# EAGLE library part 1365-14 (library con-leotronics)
DUAL ROW STRAIGHT HEADER 1364 SERIES. 1.27mm x 1.27mm. Without Fixing Post. SMT Source: http://www.leotronics.co.uk/Conexcon/Data%20Sheets/sec.%20A/1364ing.pdf
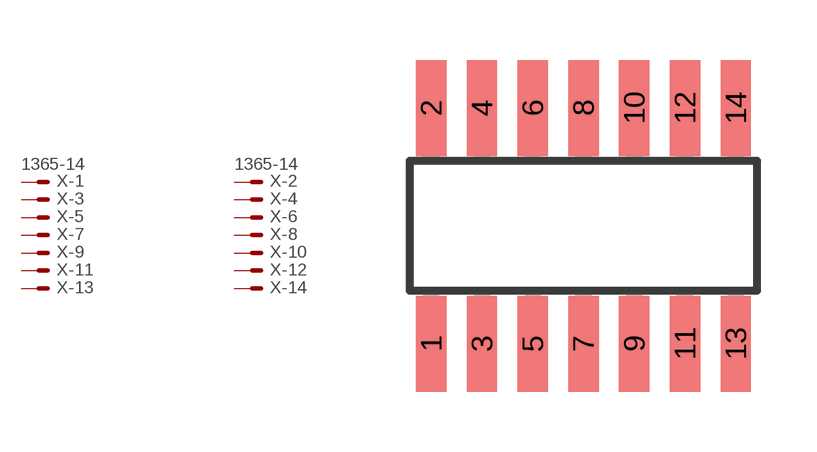
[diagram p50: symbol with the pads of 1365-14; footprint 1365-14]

Designator prefix X; gates -1=MVAL -2=MVAL -3=M -4=M -5=M -6=M -7=M -8=M -9=M -10=M -11=M -12=M -13=M -14=M

## 1365-14 (OC_FARNELL: unknown; OC_NEWARK: unknown)  [1365-14]
1  -1:S  pas
2  -2:S  pas
3  -3:S  pas
4  -4:S  pas
5  -5:S  pas
6  -6:S  pas
7  -7:S  pas
8  -8:S  pas
9  -9:S  pas
10  -10:S  pas
11  -11:S  pas
12  -12:S  pas
13  -13:S  pas
14  -14:S  pas

## Footprint 1365-14 (pad centres in mm)
DUAL ROW STRAIGHT HEADER 1364 SERIES. 1.27mm x 1.27mm. Without Fixing Post. SMT Source: http://www.leotronics.co.uk/Conexcon/Data%20Sheets/sec.%20A/1364ing.pdf
smd 0.76 x 2.4: 1 -3.81,-2.95; 2 -3.81,2.95; 3 -2.54,-2.95; 4 -2.54,2.95; 5 -1.27,-2.95; 6 -1.27,2.95; 7 0,-2.95; 8 0,2.95; 9 1.27,-2.95; 10 1.27,2.95; 11 2.54,-2.95; 12 2.54,2.95; 13 3.81,-2.95; 14 3.81,2.95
